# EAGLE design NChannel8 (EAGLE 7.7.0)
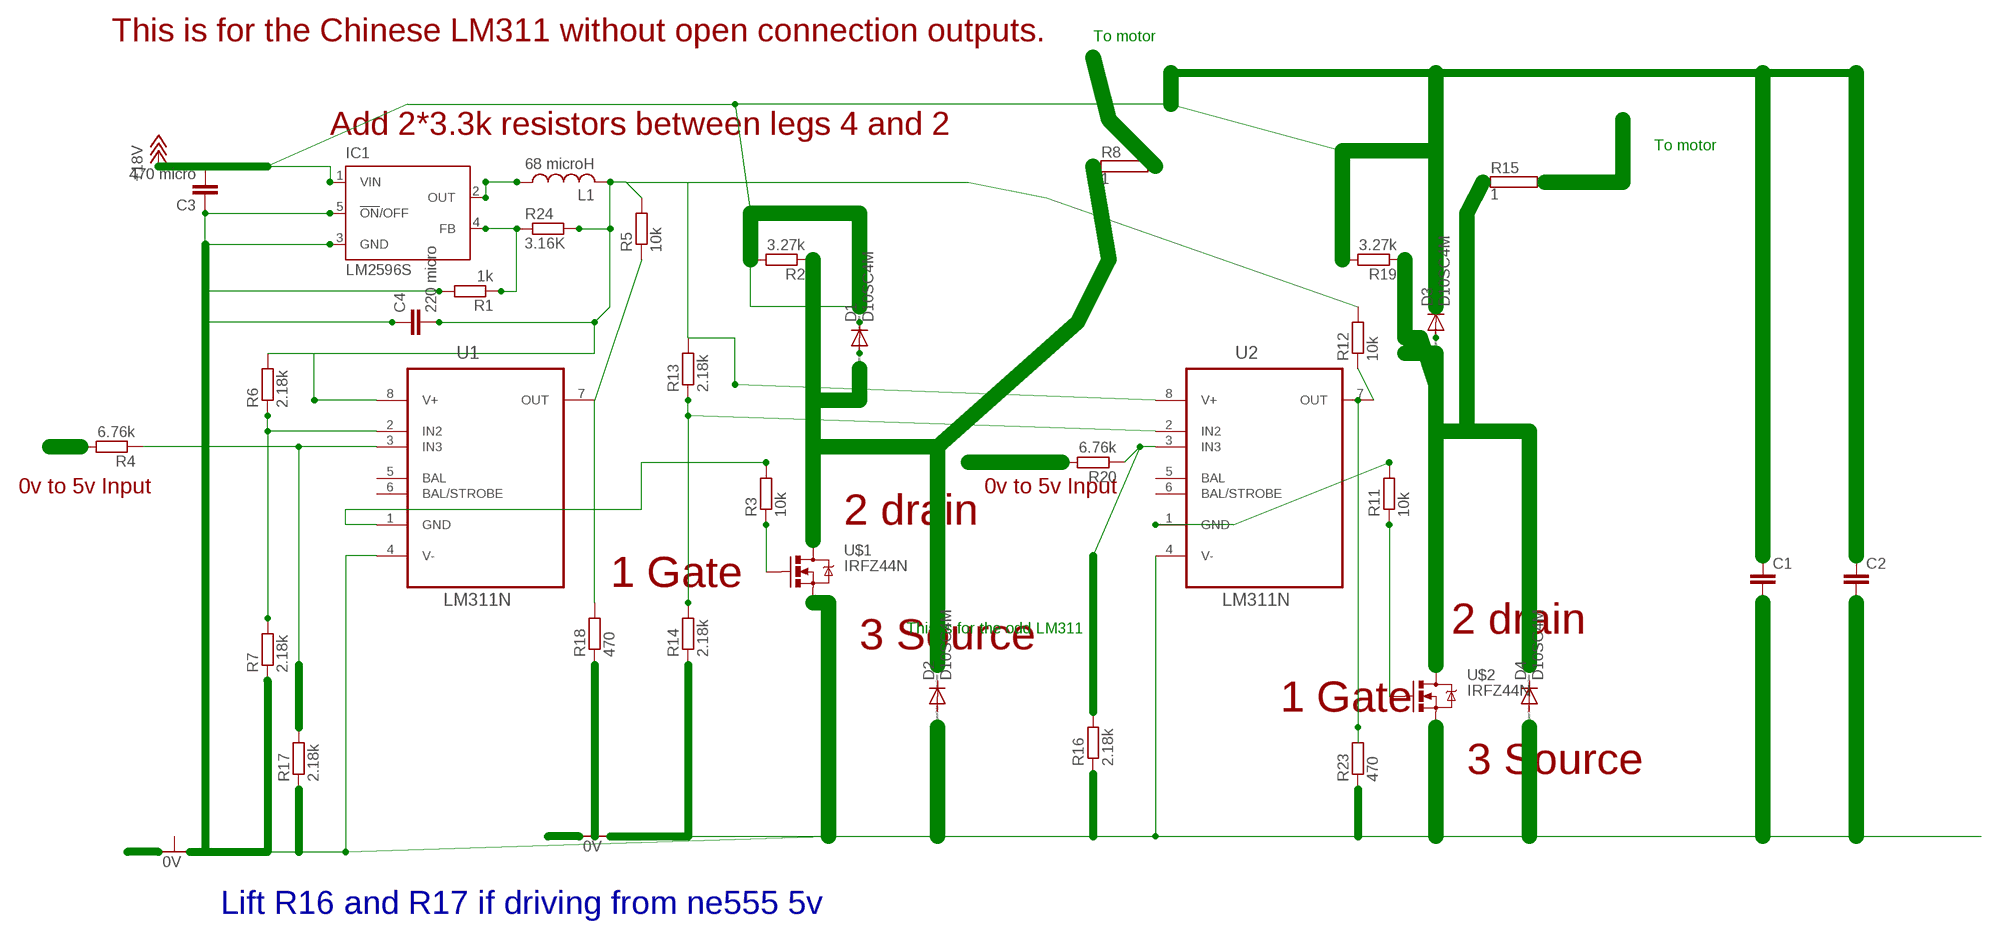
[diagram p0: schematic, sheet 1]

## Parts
C1  C-EU050H075X075  [C050H075X075]
C2  C-EU050H075X075  [C050H075X075]
C3  470 micro  C-EU050H075X075  [C050H075X075]
C4  220 micro  C-EU050H075X075  [C050H075X075]
D1  D10SC4M  BYV36  [SOD57-10]
D2  D10SC4M  BYV36  [SOD57-10]
D3  D10SC4M  BYV36  [SOD57-10]
D4  D10SC4M  BYV36  [SOD57-10]
IC1  LM2596S  [TO263-5]
L1  68 microH  L-US0204/5  [0204/5]
R1  1k  R-EU_0207/10  [0207/10]
R2  3.27k  R-EU_0207/10  [0207/10]
R3  10k  R-EU_0207/10  [0207/10]
R4  6.76k  R-EU_0207/10  [0207/10]
R5  10k  R-EU_0207/10  [0207/10]
R6  2.18k  R-EU_0207/10  [0207/10]
R7  2.18k  R-EU_0207/10  [0207/10]
R8  1  RMG100-H  [TO-247-2H]
R11  10k  R-EU_0207/10  [0207/10]
R12  10k  R-EU_0207/10  [0207/10]
R13  2.18k  R-EU_0207/10  [0207/10]
R14  2.18k  R-EU_0207/10  [0207/10]
R15  1  RMG100-H  [TO-247-2H]
R16  2.18k  R-EU_0207/10  [0207/10]
R17  2.18k  R-EU_0207/10  [0207/10]
R18  470  R-EU_0207/10  [0207/10]
R19  3.27k  R-EU_0207/10  [0207/10]
R20  6.76k  R-EU_0207/10  [0207/10]
R23  470  R-EU_0207/10  [0207/10]
R24  3.16K  R-EU_0207/10  [0207/10]
U1  LM311N  [DIP254P762X508-8]
U2  LM311N  [DIP254P762X508-8]
U$1  IRFZ44N  [TO-220]
U$2  IRFZ44N  [TO-220]

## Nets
+18V: C1.1 C2.1 C3.2 IC1.1(VIN) R2.2 R19.2
N$1: R8.2
N$2: R3.2 U1.1(GND)
N$4: R3.1 U$1.1(G)
N$5: R5.1 R18.2 U1.7(OUT)
N$6: D1.A
N$7: R2.1 R8.1 U$1.2(D)
N$8: R6.1 R7.2 U1.2(IN2)
N$9: C3.1 C4.1 IC1.3(GND) IC1.5(!ON!/OFF) R1.2 R7.1 R17.1 U1.4(V-) U$1.3(S)
N$10: R4.1 R17.2 U1.3(IN3)
N$11: IC1.2(OUT) L1.1
N$12: D1.C
N$13: R11.1 U$2.1(G)
N$14: R13.1 R14.2 R23.2 U2.2(IN2)
N$15: R16.2 R20.1 U2.3(IN3)
N$16: C1.2 C2.2 R14.1 R15.1 R16.1 R19.1 R23.1 U2.4(V-) U$2.2(D) U$2.3(S)
N$17: R4.2
N$19: R18.1
N$20: R20.2
N$21: IC1.4(FB) R1.1 R24.1
N$22: R15.2
N$23: R11.2 U2.1(GND)
N$24: R12.1 U2.7(OUT)
N$25: D3.A
N$26: D3.C
N$27: C4.2 L1.2 R5.2 R6.2 R12.2 R13.2 R24.2 U1.8(V+) U2.8(V+)
Unconnected: D2.A D2.C D4.A D4.C U1.5(BAL) U1.6(BAL/STROBE) U2.5(BAL) U2.6(BAL/STROBE)

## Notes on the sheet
- This is for the Chinese LM311 without open connection outputs. | To motor
- Add 2*3.3k resistors between legs 4 and 2
- To motor
- 0v to 5v Input | 0v to 5v Input
- 2 drain
- 1 Gate
- This is for the odd LM311 | 2 drain
- 3 Source
- 1 Gate
- 3 Source
- Lift R16 and R17 if driving from ne555 5v

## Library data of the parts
C1-C4 = rcl:C-EU: CAPACITOR, European symbol
D1-D4 = diode:BYV36: DIODE
IC1 = national-semiconductor:LM2596: SIMPLE SWITCHER® Power Converter 150 kHz 3A Step-Down Voltage Regulator Source: http://www.national.com/ds/LM/LM2596.pdf; MF: NATIONAL SEMICONDUCTOR; MPN: LM2596S-ADJ/NOPB; OC_FARNELL: 9494367; OC_NEWARK: 41K3842
L1 = resistor:L-US: INDUCTOR, American symbol
R1-R7 R11-R14 R16-R20 R23 R24 = rcl:R-EU_: RESISTOR, European symbol
R8 R15 = resistor-power:RMG100: TO-247 Power Resistor - RMG 100 Series; OC_FARNELL: unknown; OC_NEWARK: unknown
U1 U2 = NSC_By_element14_Batch_1.1:LM311N: Voltage Comparator; MPN: LM311N; OC_FARNELL: 9487220; OC_NEWARK: 07B6414; PACKAGE: DIP-8; SUPPLIER: NationalSemiconductor
U$1 U$2 = Steve:IRFZ44N

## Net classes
0 default: clearance 0.205 mm

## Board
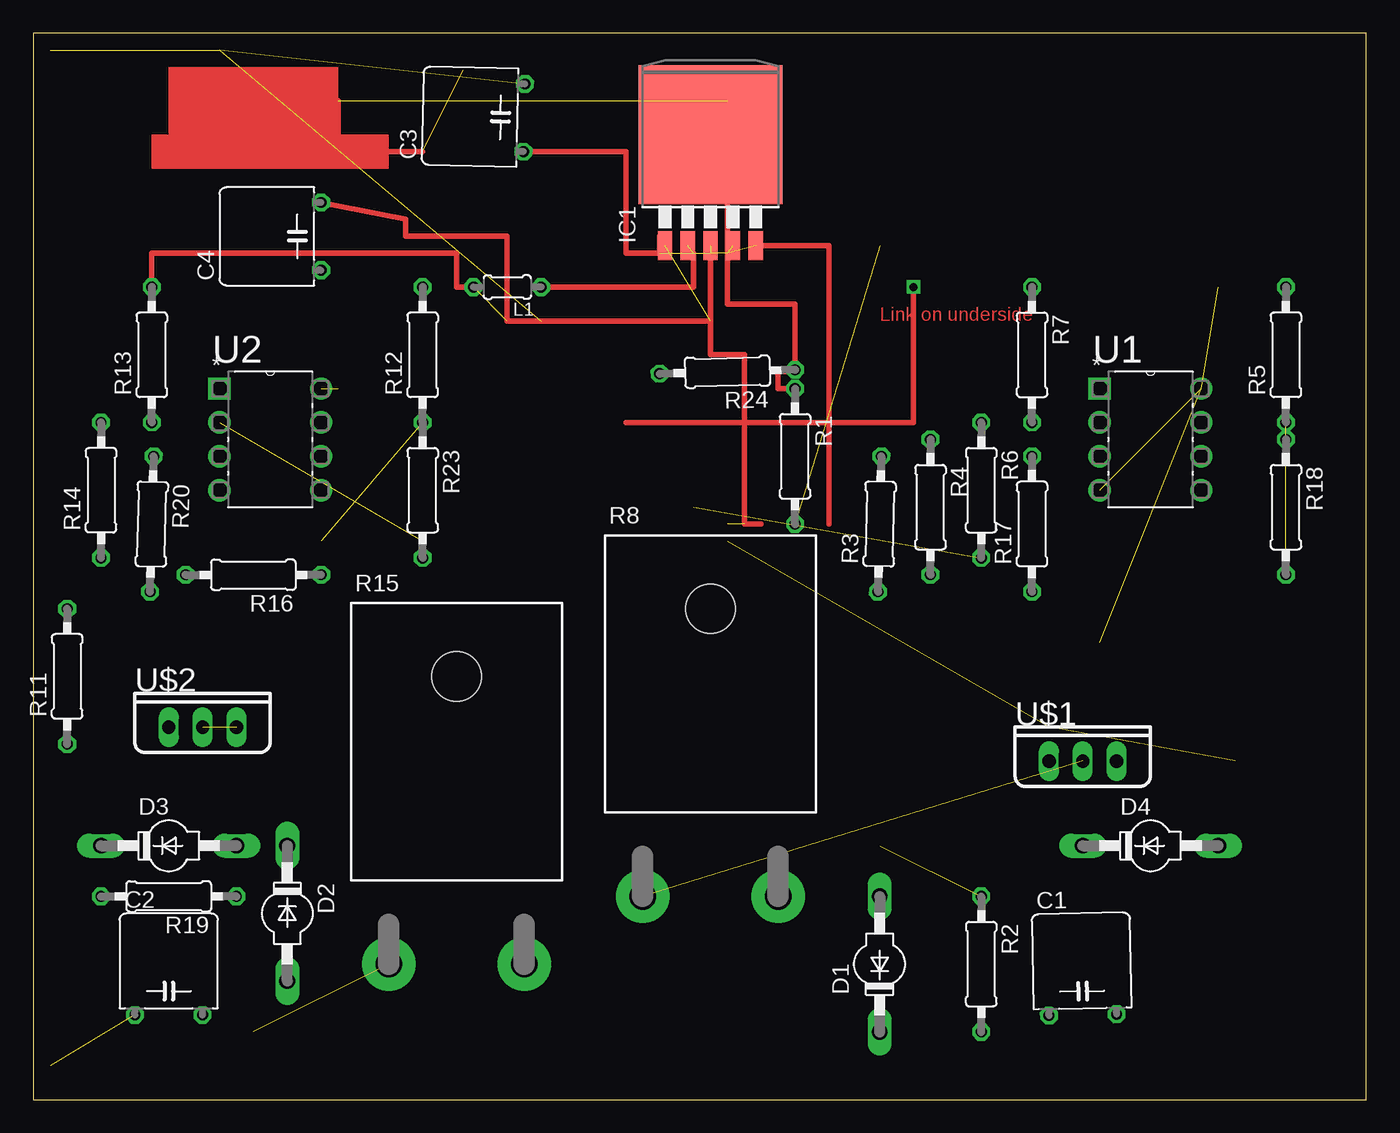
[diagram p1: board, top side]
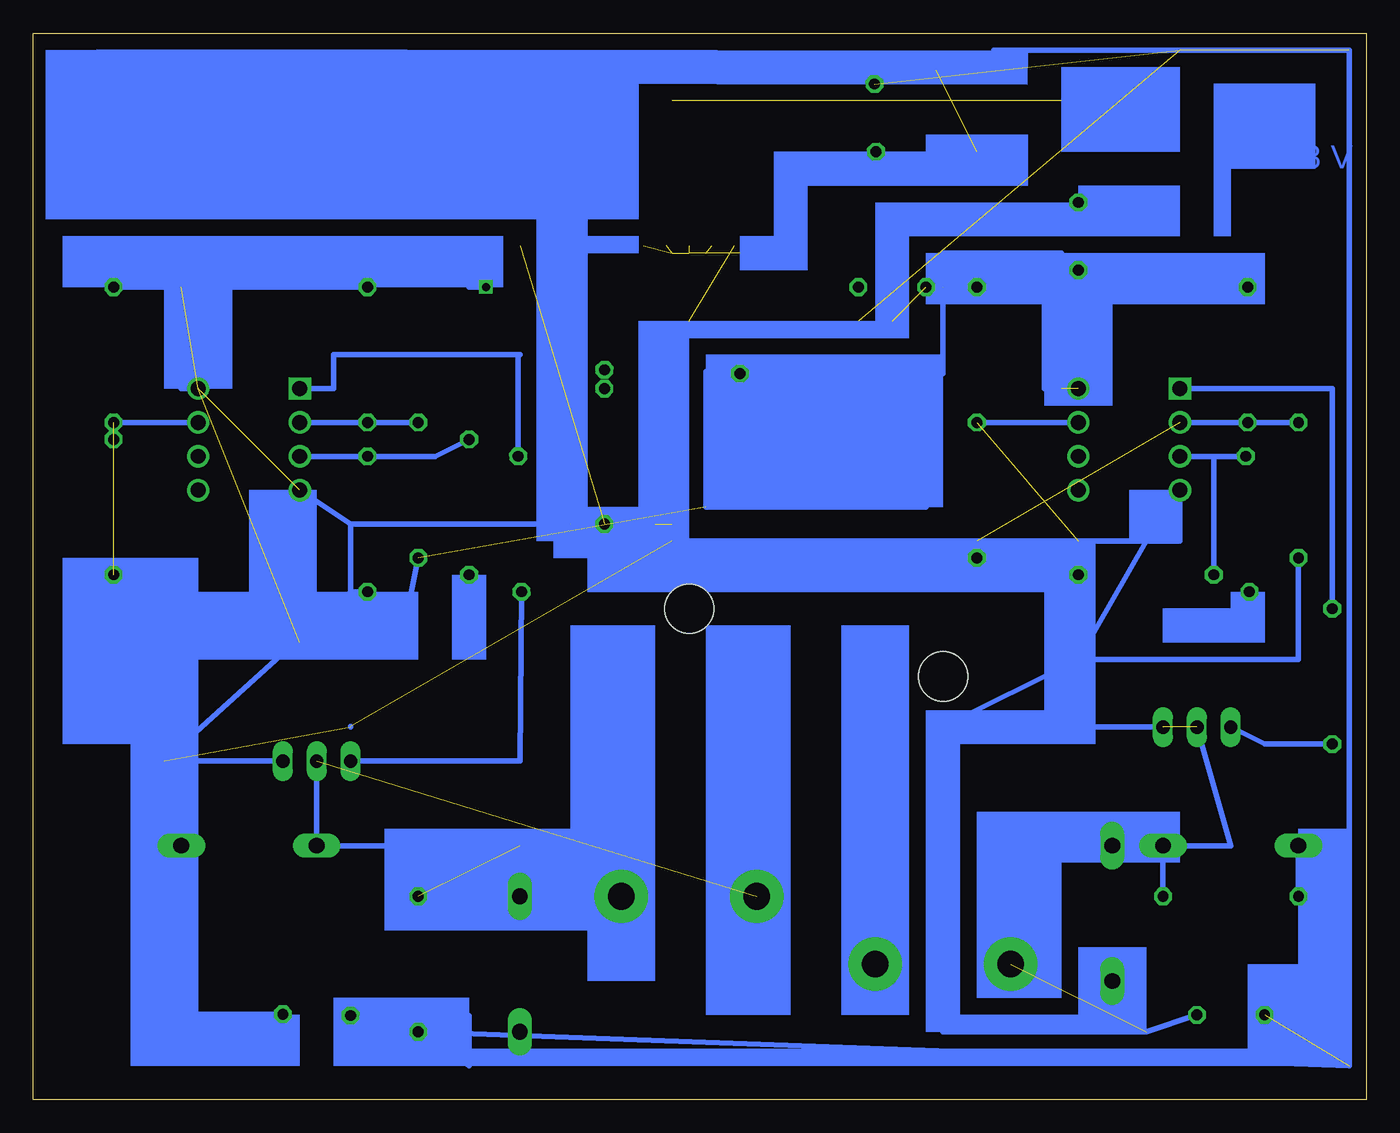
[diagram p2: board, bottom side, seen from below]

Size 100 x 80 mm. Coordinates in mm from the lower left corner, seen from the top.
Outline: 0,0 100,0 100,80 0,80 0,0
Copper layers (1*16): Top 0.035mm / dielectric 1.5mm / Bottom 0.035mm
Design rules "default": minimum track width 10mil, minimum drill 24mil, track to track 8mil, track to pad 8mil, pad to pad 8mil, via to via 8mil, smd to smd 8mil, copper to edge 40mil, drill to drill 8mil, minimum pad ring 10mil, minimum via ring 8mil, stop-mask expansion 4mil, vias tented up to drill 0mil, thermal gap 10mil

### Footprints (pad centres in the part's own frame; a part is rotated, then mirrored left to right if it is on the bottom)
C050H075X075 = drill 0.813 octagon: 1 -2.54,0; 2 2.54,0
SOD57-10 = drill 1.194 long: A 5.08,0; C -5.08,0
TO263-5 = smd 1.067 x 2.159: 1 -3.404,-5.791; 2 -1.702,-5.791; 3 0,-5.791; 4 1.702,-5.791; 5 3.404,-5.791 | smd 10.8 x 10.41: 6 0,2.54
0204/5 = drill 0.813 octagon: 1 -2.54,0; 2 2.54,0
0207/10 = drill 0.813 octagon: 1 -5.08,0; 2 5.08,0
TO-247-2H = drill 2 pad 4: 1 -5.08,-21.59; 2 5.08,-21.59 | hole 3.7: 0,0
DIP254P762X508-8 = drill 1.118 square: 1 -7.62,7.62 | drill 1.118: 2 -7.62,5.08; 3 -7.62,2.54; 4 -7.62,0; 5 0,0; 6 0,2.54; 7 0,5.08; 8 0,7.62
TO-220 = drill 1 long: 1 -2.54,0; 2 0,0; 3 2.54,0

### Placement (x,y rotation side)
C1  78.74,6.35 1.2 top
C2  10.16,6.35 0 top
C3  36.83,73.66 88.7 top
C4  21.59,64.77 90 top
D1  63.5,10.16 90 top
D2  19.05,13.97 270 top
D3  10.16,19.05 0 top
D4  83.82,19.05 0 top
IC1  50.8,69.85 0 top
L1  35.56,60.96 180 top
R1  57.15,48.26 270 top
R2  71.12,10.16 270 top
R3  63.5,43.18 88.6 top
R4  67.31,44.45 270 top
R5  93.98,55.88 90 top
R6  71.12,45.72 270 top
R7  74.93,55.88 270 top
R8  50.8,36.83 0 top
R11  2.54,31.75 90 top
R12  29.21,55.88 90 top
R13  8.89,55.88 90 top
R14  5.08,45.72 90 top
R15  31.75,31.75 0 top
R16  16.51,39.37 180 top
R17  74.93,43.18 90 top
R18  93.98,44.45 270 top
R19  10.16,15.24 180 top
R20  8.89,43.18 268.5 top
R23  29.21,45.72 270 top
R24  52.07,54.61 181.6 top
U1  87.63,45.72 0 top
U2  21.59,45.72 0 top
U$1  78.74,25.4 0 top
U$2  12.7,27.94 0 top

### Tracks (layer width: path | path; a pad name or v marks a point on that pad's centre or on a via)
+18V  (5 unrouted)
  Top 0.406: 38.1,58.42 50.8,58.42
  Bottom 0.406: C1.1 67.31,6.3 67.31,2.54 R2.2 1.27,2.54 1.27,19.05 | 1.27,19.05 1.27,78.74 27.94,78.74 | R19.2 5.08,19.05 1.27,19.05
N$2
  Bottom 0.406: U1.1 77.47,53.34 77.47,55.88 63.62,55.88 | 63.5,55.88 63.62,55.88 | 63.62,55.88 R3.2
N$3  (via drill 0.6)
  Top 0.406: v66.04,60.96 66.04,50.8 44.45,50.8
  Bottom 0.406: 67.31,60.96 v66.04,60.96
N$4
  Bottom 0.406: U$1.1 63.5,25.4 R3.1
N$5  (1 unrouted)
  Bottom 0.406: R5.1 U1.7
N$7  (2 unrouted)
  Bottom 0.406: U$1.2 78.74,19.05 63.5,19.05
N$8
  Bottom 0.406: R6.1 R7.2 U1.2
N$9  (10 unrouted)
  Top 0.406: 54.61,43.18 53.34,43.18 53.34,55.88 50.8,55.88 50.8,63.5 | C3.1 44.45,71.12 44.45,63.5 46.99,63.5 46.99,64.77 | 22.86,74.93 22.86,71.12 29.21,71.12 | 52.07,74.93 52.07,63.5 | IC1.5 59.69,64.06 59.69,43.18
  Bottom 0.406: U1.4 76.2,43.18 | 76.2,43.18 52.07,43.18 | U$1.3 90.17,25.4 76.2,38.1 | 76.2,38.1 76.2,43.18 | R17.1 76.2,38.1 | R7.1 88.9,60.96 88.9,53.34 87.63,53.34 | C4.1 29.21,62.23 29.21,60.96
N$10
  Bottom 0.406: U1.3 R17.2 69.85,48.26 R4.1
N$11  (1 unrouted)
  Top 0.406: L1.1 49.53,60.96 49.53,63.5
N$13
  Bottom 0.406: R11.1 7.62,26.67 U$2.1
N$14  (1 unrouted)
  Bottom 0.406: U2.2 R13.1 R14.2 | R23.2 29.21,41.91
N$15
  Bottom 0.406: R16.2 11.43,48.26 | U2.3 11.43,48.26 | R20.1 11.43,48.26
N$16  (5 unrouted)
  Bottom 0.406: U2.4 13.97,41.91 16.51,41.91 | 16.51,41.91 21.59,41.91 | 21.59,41.91 52.07,41.91 52.07,43.18 | U$2.3 31.75,27.94 | 31.75,27.94 31.75,5.08 16.51,5.08 C2.2 | 31.75,27.94 21.59,33.02 | 21.59,33.02 16.51,41.91 | 76.2,27.99 76.2,27.94 | R16.1 21.59,41.91 | R14.1 5.08,33.02 21.59,33.02 | C1.2 90.17,6.4 90.17,25.4 | R19.1 15.24,19.05 10.16,19.05 U$2.2
N$21  (1 unrouted)
  Top 0.406: R1.1 55.88,53.34 55.88,54.61 57.15,54.61 R24.1 57.15,59.69 52.07,59.69 52.07,63.5
N$23
  Bottom 0.406: R11.2 2.54,53.34 U2.1
N$24
  Bottom 0.406: R12.1 U2.7
N$27  (6 unrouted)
  Top 0.406: C4.2 27.94,66.04 27.94,64.77 35.56,64.77 35.56,58.42 38.1,58.42 | L1.2 31.75,60.96 31.75,63.5 8.89,63.5 R13.2
  Bottom 0.406: R6.2 72.39,34.29 80.01,34.29 | R5.2 88.9,60.96 | R12.2 24.13,60.96 24.13,53.34 22.86,53.34 22.86,63.5 31.75,63.5 31.75,60.96 31.75,54.61 | 31.75,54.61 33.02,54.61 | 33.02,54.61 49.53,54.61 49.53,44.45 33.02,44.45 33.02,54.61 | R24.2 31.75,54.47 31.75,54.61
(copper drawn outside any net)
  shapes: Bottom area x55, Top area x2

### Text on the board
Top: Link on underside
Bottom: +18 V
